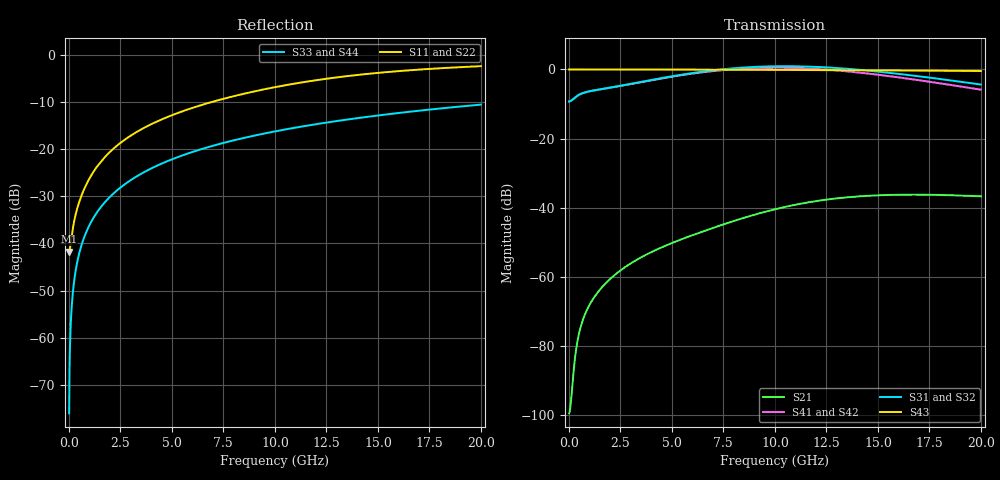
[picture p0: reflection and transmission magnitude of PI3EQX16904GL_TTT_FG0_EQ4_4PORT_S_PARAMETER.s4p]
! NPort=4 DATA=2000 NOISE=0 GROUPDELAY=0 COMPLEX_DATAFORMAT=POLAR
! NumOfBlock=1 NumOfParam=0
! .MODEL Smodel S TSTONEFILE=PI3EQX16904GL_TTT_FG0_EQ4_4PORT_S_PARAMETER.s4p TYPE=S
!  -- The above .MODEL line can be used for the S element in the netlist.
! The s parameter is extracted from the linear redriver, it is not bi-directional; only s(4,1)s(4,2) and s(3,1)s(3,2)
! should be the insertion loss
!Port definition:
!Port1 = input+
!Port2 = input-
!Port3 = output+
!Port4 = output-
# Hz S MA R  50
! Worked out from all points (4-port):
!   2000 points, 10 MHz to 20 GHz, reference 50 ohm
!   strongest paths, dB at 10 MHz, 5.01 GHz, 10.01 GHz, 15.01 GHz, 20 GHz:
!     S43: 0.0, 0.0, -0.1, -0.3, -0.4
!     S31: -9.2, -2.0, 0.9, -0.6, -4.4
!     S32: -9.2, -2.1, 0.6, -1.0, -4.7
!     S41: -9.2, -2.1, 0.5, -1.5, -5.8
!     S42: -9.2, -2.2, 0.2, -1.9, -6.2
!     S21: -99.6, -50.2, -40.5, -36.4, -36.7
!   lowest |S11| = -41.7 dB at 10 MHz (marker M1), VSWR 1.02, Z = 49.2 - j0.0603 ohm
!   |S11| at or under -10 dB: start of sweep to 6.893 GHz
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1e7  0.008182 -175.7  1.05e-05 7.7  0 0.0  0 0.0
     1.05e-05 7.7  0.008182 -175.7  0 0.0  0 0.0
     0.3452 0.4  0.3452 -179.6  0.0001571 -90.0  1 -0.0
     0.3452 -179.6  0.3452 0.4  1 -0.0  0.0001571 -90.0
2e8  0.01483 -130.6  3.431e-05 106.2  0 0.0  0 0.0
     3.431e-05 106.2  0.01483 -130.6  0 0.0  0 0.0
     0.3715 8.0  0.3714 -172.1  0.003142 -90.2  1 -0.2
     0.3715 -172.4  0.3713 7.5  1 -0.2  0.003142 -90.2
6.2e8  0.03268 -112.4  0.0002097 114.5  0 0.0  0 0.0
       0.0002097 114.5  0.03268 -112.4  0 0.0  0 0.0
       0.449 8.7  0.4485 -171.6  0.009738 -90.6  0.9999 -0.6
       0.4489 -172.4  0.4484 7.3  0.9999 -0.6  0.009738 -90.6
2.97e9  0.1383 -101.5  0.001537 101.0  0 0.0  0 0.0
        0.001536 100.9  0.1383 -101.6  0 0.0  0 0.0
        0.6166 -6.2  0.6111 172.7  0.0466 -92.8  0.9988 -2.7
        0.6138 168.4  0.6084 -12.6  0.9988 -2.7  0.0466 -92.8
1.002e10  0.4579 -112.9  0.009585 60.3  0 0.0  0 0.0
          0.009486 61.0  0.4574 -112.9  0 0.0  0 0.0
          1.115 -98.4  1.077 80.6  0.1553 -99.3  0.9869 -8.9
          1.061 64.1  1.025 -116.9  0.9869 -8.9  0.1553 -99.3
1.418e10  0.6223 -123.3  0.01473 17.1  0 0.0  0 0.0
          0.01462 18.3  0.6215 -123.3  0 0.0  0 0.0
          0.9848 -162.8  0.9474 16.4  0.217 -103.0  0.9742 -12.5
          0.8966 -6.7  0.8626 172.5  0.9742 -12.5  0.217 -103.0
2e10  0.7645 -136.0  0.01459 -33.3  0 0.0  0 0.0
      0.01457 -31.5  0.7643 -136.0  0 0.0  0 0.0
      0.6057 121.5  0.5801 -59.1  0.2986 -108.1  0.9506 -17.4
      0.51 -90.5  0.4885 88.9  0.9506 -17.4  0.2986 -108.1
